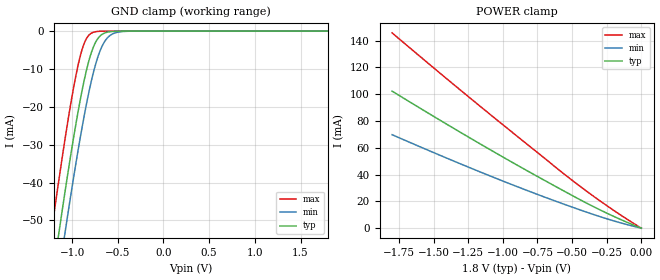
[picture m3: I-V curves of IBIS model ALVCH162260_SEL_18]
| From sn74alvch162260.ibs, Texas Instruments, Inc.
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[Model]   ALVCH162260_SEL_18
Model_type  Input
Vinl=0.5775
Vinh=1.2675
| variable   typ   min   max
C_comp   26.37pF   21.86pF   32.81pF
[Temperature Range]   40   100   -40
| Ambient temperature   25   85   -40
[Voltage range]   1.8   1.65   1.95
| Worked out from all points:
|   GND clamp passes 1 mA (typ) near -0.68 V on its own axis
|   POWER clamp passes 1 mA (typ) near -0.02 V on its own axis
[GND Clamp]
| ALVCH162260_SEL_18
|   Voltage   I(typ)   I(min)   I(max)
-1.8V     -169.5mA   -179.7mA   -156.7mA
-1.245V   -70.18mA   -81.02mA   -56.25mA
-1.22V    -65.92mA   -76.78mA   -51.96mA
-1.14V    -52.55mA   -63.42mA   -38.55mA
-1.075V   -42.06mA   -52.87mA   -28.16mA
-920mV    -19.37mA   -29.44mA   -7.486mA
-860mV    -12.16mA   -21.41mA   -2.808mA
-795mV    -6.112mA   -13.8mA    -645.2uA
-730mV    -2.404mA   -7.745mA   -117.8uA
-660mV    -692.8uA   -3.429mA   -17.66uA
-495mV    -25.94uA   -271uA     -195.5nA
1.8V      1.111nA    770.5nA    2.881pA
[POWER Clamp]
| ALVCH162260_SEL_18
|   Voltage   I(typ)   I(min)   I(max)
-1.8V     102.3mA    69.75mA    145.7mA
-1.12V    60.25mA    40.13mA    87.25mA
-540mV    26.68mA    17.21mA    38.97mA
-270mV    12.23mA    7.675mA    18.31mA
-16.28fV  57.05pA    185.2pA    36.47pA
